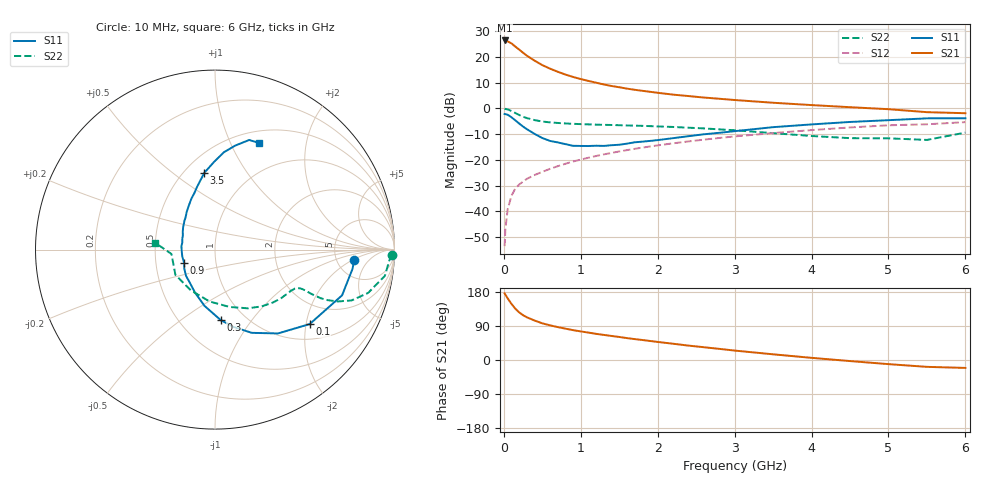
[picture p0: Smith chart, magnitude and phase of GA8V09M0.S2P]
! Infineon Technologies  Discrete & RF Semiconductors
! BF775
! Si NPN RF Bipolar Junction Transistor in SOT23
! VCE = 8 V  IC = 9 mA
! Common Emitter S-Parameters:  May  1996
# GHz  S  MA  R  50
!  f  S11  S21  S12  S22
! GHz  MAG  ANG  MAG  ANG  MAG  ANG  MAG  ANG
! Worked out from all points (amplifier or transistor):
!   36 points, 10 MHz to 6 GHz, reference 50 ohm
!   highest |S21| = 26.4 dB at 10 MHz (marker M1)
!   |S21| within 3 dB of that: start of sweep to 175.8 MHz
!   unconditionally stable (mu >= 1): 667.3 MHz to 2.888 GHz
!   at 250 MHz: K = 0.63, MSG = 25.0 dB, |S12| = -28.5 dB
!   at 1.4 GHz: K = 1.10, MAG = 11.1 dB, |S12| = -17.3 dB
!   at 6 GHz: K = 0.89, MSG = 1.7 dB, |S12| = -5.3 dB
!   S11 on the Smith chart (normalised r, x): 10 MHz: 7.41, -2.09; 100 MHz: 1.39, -2.10; 300 MHz: 0.77, -0.72; 900 MHz: 0.70, -0.11; 3.5 GHz: 0.62, +0.65; 6 GHz: 0.64, +1.29
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0.01  0.778 -4.1  20.88 175.9  0.0021 91.3  0.9881 -1.7
0.02  0.7736 -8.0  20.49 172.4  0.0045 88.1  0.9729 -3.6
0.05  0.7525 -19.8  20.05 162.7  0.011 81.6  0.9576 -8.8
0.1  0.6711 -38.2  18.27 147.8  0.0202 72.3  0.8866 -15.8
0.15  0.5841 -53.1  15.83 135.2  0.0278 67.6  0.812 -20.4
0.2  0.5069 -66.2  13.86 125.6  0.0332 64.1  0.7429 -22.9
0.25  0.443 -76.5  12.05 118.2  0.0378 62.6  0.6865 -24.2
0.3  0.3938 -85.4  10.55 112.6  0.0428 62.6  0.6474 -24.7
0.4  0.3192 -100.5  8.446 104.1  0.0507 62.5  0.5917 -24.7
0.5  0.2653 -114.6  6.932 96.8  0.0584 63.3  0.5555 -24.4
0.6  0.233 -126.6  5.918 91.5  0.0668 64.0  0.5344 -24.3
0.7  0.2181 -137.7  5.154 86.9  0.0752 64.8  0.5207 -24.5
0.9  0.1873 -157.1  4.081 78.8  0.0928 64.8  0.5012 -25.4
1.1  0.1855 -176.4  3.413 72.3  0.1099 64.9  0.4889 -27.2
1.3  0.1864 168.1  2.915 66.2  0.1276 64.2  0.4786 -29.2
1.6  0.2064 150.5  2.421 57.8  0.1544 62.4  0.4653 -33.2
2.2  0.2636 126.6  1.851 42.9  0.2093 58.0  0.4352 -43.0
3  0.3604 106.4  1.454 24.9  0.285 50.3  0.3759 -60.5
3.5  0.4314 98.0  1.286 15.0  0.3311 44.6  0.3299 -75.7
4.5  0.5445 84.8  1.054 -2.8  0.426 32.4  0.2638 -120.8
5.5  0.6398 72.7  0.844 -18.1  0.4908 17.3  0.2438 -174.3
6  0.6428 67.5  0.805 -20.9  0.5406 13.2  0.3383 173.3
